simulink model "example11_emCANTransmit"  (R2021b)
settings: Solver=FixedStepAuto  StartTime=0  StopTime=inf  FixedStep=0.5  RelTol=1e-3  EnableMultiTasking=on
undefined symbols (not defined in the file or in its folder): based, Big, bool, classic, dsPic33, Endian, Little, MCC, Microchip, PIC24
libraries: embeddedCreatorLib x8, emCANLib x6, emMBSlaveLib x1

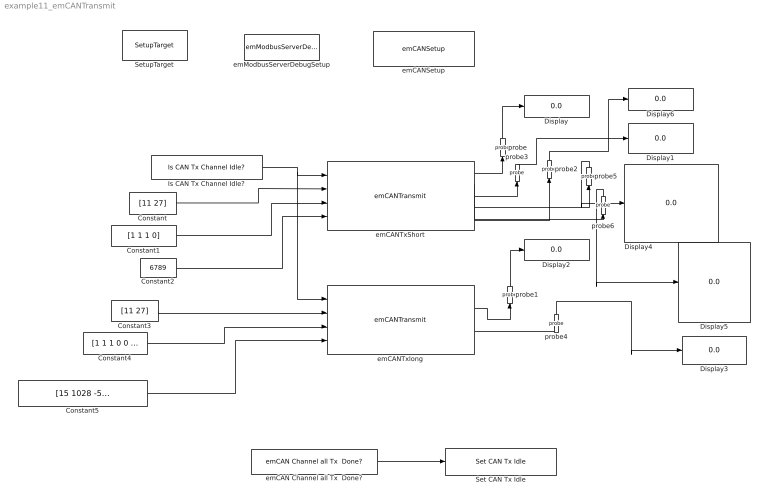
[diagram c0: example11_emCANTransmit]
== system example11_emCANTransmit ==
  Constant : Constant  Value=[11 27]  OutDataTypeStr=int8
  Constant1 : Constant  Value=[1 1 1 0]  OutDataTypeStr=boolean
  Constant2 : Constant  Value=6789  OutDataTypeStr=int32
  Constant3 : Constant  Value=[11 27]  OutDataTypeStr=int8
  Constant4 : Constant  Value=[1 1 1 0 0 1]  OutDataTypeStr=boolean
  Constant5 : Constant  Value=[15 1028 -5899]  OutDataTypeStr=int16
  Display{,1..6} (7 alike) : Display
  Is CAN Tx Channel Idle? : emCANLib/Is CAN Tx Channel Idle?  Tag=isCANTx_Idle  c_CAN_DeviceNo=1  c_ChannelName=Channel A  c_sampleTime=-1
  Set CAN Tx Idle : emCANLib/Set CAN Tx Idle  Tag=setCANTx2Idle  c_CAN_DeviceNo=1  c_ChannelName=Channel A
  SetupTarget : embeddedCreatorLib/SetupTarget  Tag=SetupTarget  Priority=0  c_platform=Microchip PIC24/dsPic33 based on MCC classic  c_debug=on
  emCAN Channel all Tx  Done? : emCANLib/emCAN Channel all Tx  Done?  c_CAN_DeviceNo=1  c_ChannelName=Channel A  c_sampleTime=-1
  emCANSetup : emCANLib/emCANSetup  Tag=emCANBus  c_CAN_DeviceNo=1  c_saved_SettingFormat=1  c_SettingFormat=Settings in Hex Data format  c_Mask0=7F0  c_Mask1=1FFF00FFX  c_Mask2=7F0  c_CANID_short=[120,31,50124X]  c_CANID_long=[12340112X]  c_FrameNoWay=1-based frame No  c_MaxFrameQty=2  c_enableSync=on  c_Sync_RxCANID=12340218x  c_Com_Fault_detection_Time=200  c_ASeq_QTY=31  c_BSeq_QTY=0  c_CSeq_QTY=0  c_RxStdShort_listData=49  c_RxExtShort_listData=327972  c_RxStdLong_listData=-1  c_RxExtLong_listData=305398034  c_RxStdSyncData=-1  c_RxExtSyncData=305398296  c_txChaanelA_DataLength="\"\""  c_txChaanelB_DataLength="\"\""  c_txChaanelC_DataLength="\"\""  c_sampleTime=-1
  emCANTxShort : emCANLib/emCANTransmit  Tag=emCANBUSTx  c_CAN_DeviceNo=1  c_SettingFormat="CAN ID  in Hex Data format"  c_TxChannel=Channel A  c_SeqNo=Seq0  c_TransmittedType=Standard 11 bits CAN ID short frame  c_CANID=67  c_RTR=off  c_DataType="[int8*2 bool*4 int32  ]"  c_Endian=Little-Endian  c_NeedResponse=on  c_Timeout=5000  c_ResponseCANIDType=Extended 29 bits CAN ID long frame  c_CANID_Response=12340112  c_ResposeDataType="[int8*2  bool*6 uint32*2]"  c_InputDataQty="[2  4  1]"  c_InputType="[2  8  6]"  c_OutputDataQty="[2  6  2]"  c_OutputType="[2  8  7]"  c_currentHex=on
  emCANTxlong : emCANLib/emCANTransmit  Tag=emCANBUSTx  c_CAN_DeviceNo=1  c_SettingFormat="CAN ID  in Hex Data format"  c_TxChannel=Channel A  c_SeqNo=Seq7  c_TransmittedType=Extended 29 bits CAN ID long frame  c_CANID=88  c_RTR=off  c_DataType="[int8*2 bool*6 int16*3  ]"  c_Endian=Big-Endian  c_NeedResponse=off  c_Timeout=5000  c_ResponseCANIDType=Extended 29 bits CAN ID long frame  c_CANID_Response=12340112  c_ResposeDataType="[int8*2  bool*6 uint32*2]"  c_InputDataQty="[2  6  3]"  c_InputType="[2  8  4]"  c_OutputDataQty="[2  6  2]"  c_OutputType="[2  8  7]"  c_currentHex=on
  emModbusServerDebugSetup : emMBSlaveLib/emModbusServerDebugSetup  Tag=emModbusSlaveSetup  c_objID=0  c_uartNo=2  c_baudrate=19200  c_serverID=1  c_baudrate4PC=19200  c_forceLongerSpace=on  c_holdingRegsQTY=1000  c_minHoldingAddr=789  c_inputRegsQTY=200  c_minInputRegAddr=20  c_coilRegsQTY=300  c_minCoilAddr=30  c_discreteRegsQTY=400  c_minDiscreteAddr=40  c_enableDebug=on  c_breakpointMaxQTY=100  c_probeMaxWordQTY=200  c_emWaitQTY=0  g_COMPortNo=COM5  c_Name_method=By physical port name and bit number  c_PortName=B  c_BitNo=11  c_TxEnable485="\"LATBbits.LATB11\""  c_TxEnable485Polarity=on
  probe : embeddedCreatorLib/probe  Tag=emProbe  c_ObjID=5  c_serverID=1  c_UartNo=1  c_StartAddr=16  c_ConstantDataSource=off
  probe1 : embeddedCreatorLib/probe  Tag=emProbe  c_ObjID=3  c_serverID=1  c_UartNo=1  c_StartAddr=14  c_ConstantDataSource=off
  probe2 : embeddedCreatorLib/probe  Tag=emProbe  c_ObjID=6  c_serverID=1  c_UartNo=1  c_StartAddr=17  c_ConstantDataSource=off
  probe3 : embeddedCreatorLib/probe  Tag=emProbe  c_ObjID=1  c_serverID=1  c_UartNo=1  c_StartAddr=8  c_ConstantDataSource=off
  probe4 : embeddedCreatorLib/probe  Tag=emProbe  c_ObjID=4  c_serverID=1  c_UartNo=1  c_StartAddr=15  c_ConstantDataSource=off
  probe5 : embeddedCreatorLib/probe  Tag=emProbe  c_ObjID=0  c_serverID=1  c_UartNo=1  c_StartAddr=2  c_ConstantDataSource=off
  probe6 : embeddedCreatorLib/probe  Tag=emProbe  c_ObjID=2  c_serverID=1  c_UartNo=1  c_StartAddr=10  c_ConstantDataSource=off
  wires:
  emCAN Channel all Tx  Done?/1 -> Set CAN Tx Idle/1
  Is CAN Tx Channel Idle?/1 -> emCANTxlong/1, emCANTxShort/1
  Constant/1 -> emCANTxShort/2
  Constant1/1 -> emCANTxShort/3
  Constant2/1 -> emCANTxShort/4
  emCANTxShort/1 -> probe/1
  probe/1 -> Display/1
  Constant3/1 -> emCANTxlong/2
  Constant4/1 -> emCANTxlong/3
  Constant5/1 -> emCANTxlong/4
  probe1/1 -> Display2/1
  emCANTxlong/1 -> probe1/1
  emCANTxlong/2 -> probe4/1
  probe4/1 -> Display3/1
  emCANTxShort/2 -> probe2/1
  probe2/1 -> Display6/1
  emCANTxShort/3 -> probe3/1
  probe3/1 -> Display1/1
  emCANTxShort/4 -> probe5/1
  probe5/1 -> Display4/1
  emCANTxShort/5 -> probe6/1
  probe6/1 -> Display5/1
